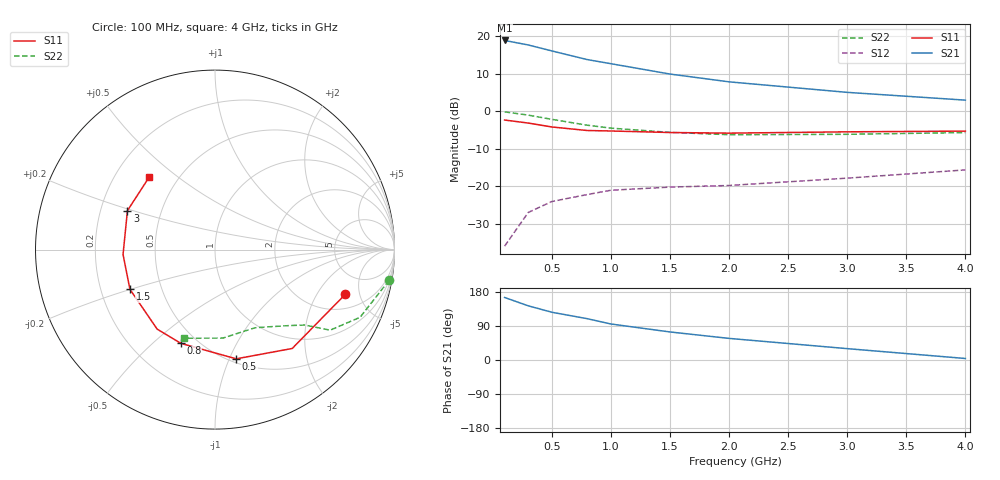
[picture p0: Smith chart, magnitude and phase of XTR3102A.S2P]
! HXTR-3102 Common Emitter
! Vce=15V Ic=20mA
# ghz s ma r 50
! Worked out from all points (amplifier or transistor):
!   9 points, 100 MHz to 4 GHz, reference 50 ohm
!   highest |S21| = 18.9 dB at 100 MHz (marker M1)
!   |S21| within 3 dB of that: start of sweep to 526.2 MHz
!   unconditionally stable (mu >= 1): 1.966 GHz to 3.239 GHz
!   at 300 MHz: K = 0.22, MSG = 22.3 dB, |S12| = -26.9 dB
!   at 1 GHz: K = 0.61, MSG = 16.9 dB, |S12| = -21.0 dB
!   at 4 GHz: K = 0.93, MSG = 9.3 dB, |S12| = -15.6 dB
!   S11 on the Smith chart (normalised r, x): 100 MHz: 2.99, -3.62; 500 MHz: 0.54, -1.06; 800 MHz: 0.41, -0.62; 1.5 GHz: 0.33, -0.20; 3 GHz: 0.32, +0.19; 4 GHz: 0.35, +0.40
0.1  0.767 -19.0  8.81 165.0  0.016 72.0  0.985 -10.0
0.3  0.699 -52.0  7.674 143.0  0.045 60.0  0.892 -25.0
0.5  0.62 -79.0  6.383 126.0  0.063 50.0  0.783 -35.0
0.8  0.556 -110.0  4.898 109.0  0.078 41.0  0.654 -40.0
1  0.548 -126.0  4.317 95.0  0.089 34.0  0.598 -45.0
1.5  0.523 -155.0  3.143 74.0  0.098 60.0  0.525 -55.0
2  0.513 -177.0  2.475 57.0  0.103 29.0  0.489 -63.0
3  0.534 156.0  1.792 30.0  0.129 31.0  0.495 -85.0
4  0.546 132.0  1.412 4.0  0.166 29.0  0.522 -109.0
